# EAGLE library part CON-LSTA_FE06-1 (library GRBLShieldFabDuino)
FEMALE HEADER
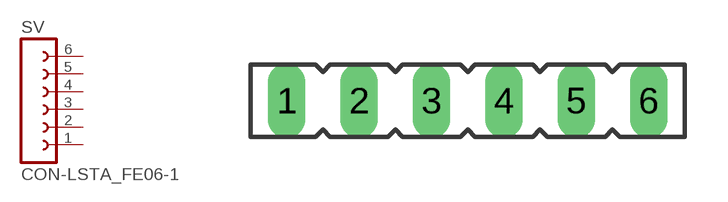
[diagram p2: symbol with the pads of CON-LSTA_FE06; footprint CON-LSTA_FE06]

Designator prefix SV

## CON-LSTA_FE06-1 (OC_FARNELL: unknown; OC_NEWARK: unknown)  [CON-LSTA_FE06]
1  1  pas
2  2  pas
3  3  pas
4  4  pas
5  5  pas
6  6  pas

## Footprint CON-LSTA_FE06 (pad centres in mm)
FEMALE HEADER
drill 0.813 long: 1 -6.35,0; 2 -3.81,0; 3 -1.27,0; 4 1.27,0; 5 3.81,0; 6 6.35,0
